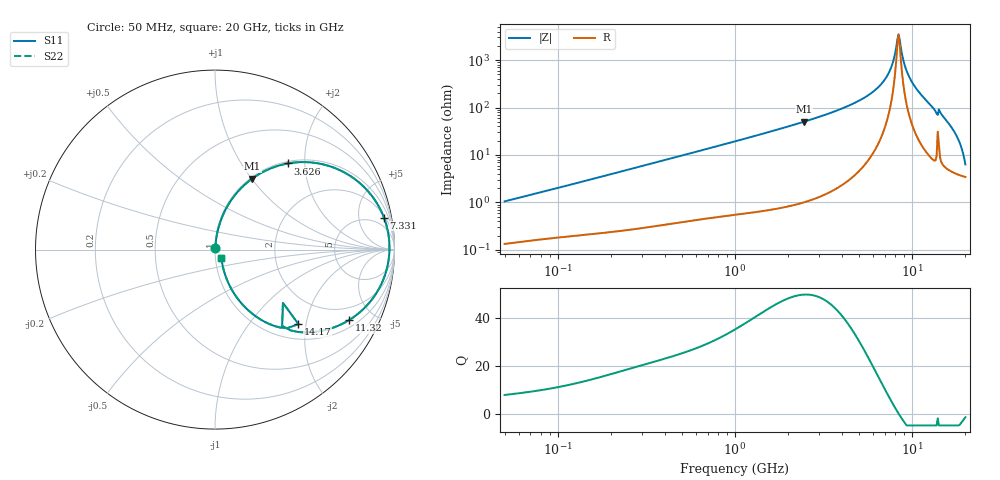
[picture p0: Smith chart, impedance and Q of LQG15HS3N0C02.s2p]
!Murata Part Number: LQG15HS3N0C02
!These Parameters are Measured in Series Mode Connection
!  o--[Z]--o
!Port1  Port2
!  o-------o
!Freq. Start=50[MHz] Stop=20[GHz], 401[Steps]
# Hz S RI R 50
!Freq.(Hz) S11(Real) S11(Imag) S21(Real) S21(Imag) S12(Real) S12(Imag) S22(Real) S22(Imag)
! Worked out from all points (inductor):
!   401 points, 50 MHz to 20 GHz, reference 50 ohm
!   read as one part in series: L = 3.28 nH near 51.52 MHz
!   highest Q = 50 at 2.456 GHz (marker M1), where L = 3.26 nH
!   self-resonance near 8.389 GHz
!   S11 on the Smith chart (normalised r, x): 50 MHz: 1.00, +0.02; 3.626 GHz: 1.04, +1.64; 7.331 GHz: 2, +10; 11.32 GHz: 1.32, -3.61; 14.17 GHz: 1.33, -1.81; 20 GHz: 1.07, -0.11
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5e7  0.00144 0.0104  0.9986 -0.0104  0.9986 -0.0104  0.00144 0.0104
1.364002e8  0.00278 0.0271  0.9972 -0.0271  0.9972 -0.0271  0.00278 0.0271
3.721004e8  0.00844 0.0718  0.9916 -0.0718  0.9916 -0.0718  0.00844 0.0718
1e9  0.0411 0.1848  0.9589 -0.1848  0.9589 -0.1848  0.0411 0.1848
2.456456e9  0.2071 0.3953  0.7929 -0.3953  0.7929 -0.3953  0.2071 0.3953
2.728004e9  0.2494 0.4228  0.7506 -0.4228  0.7506 -0.4228  0.2494 0.4228
3.626126e9  0.4047 0.4798  0.5953 -0.4798  0.5953 -0.4798  0.4047 0.4798
5.683258e9  0.7628 0.4044  0.2372 -0.4044  0.2372 -0.4044  0.7628 0.4044
6.601595e9  0.8802 0.2909  0.1198 -0.2909  0.1198 -0.2909  0.8802 0.2909
7.331367e9  0.9412 0.1784  0.0588 -0.1784  0.0588 -0.1784  0.9412 0.1784
7.442007e9  0.9477 0.1603  0.0523 -0.1603  0.0523 -0.1603  0.9477 0.1603
7.784049e9  0.9629 0.103  0.0371 -0.103  0.0371 -0.103  0.9629 0.103
8.264682e9  0.9719 0.0212  0.0281 -0.0212  0.0281 -0.0212  0.9719 0.0212
8.389408e9  0.972 2.59e-05  0.028 -2.59e-05  0.028 -2.59e-05  0.972 2.59e-05
9.457416e9  0.9353 -0.1731  0.0647 0.1731  0.0647 0.1731  0.9353 -0.1731
1.131968e10  0.7481 -0.3921  0.2519 0.3921  0.2519 0.3921  0.7481 -0.3921
1.295331e10  0.5202 -0.4612  0.4798 0.4612  0.4798 0.4612  0.5202 -0.4612
1.417136e10  0.4647 -0.4148  0.5353 0.4148  0.5353 0.4148  0.4647 -0.4148
1.504638e10  0.3034 -0.415  0.6966 0.415  0.6966 0.415  0.3034 -0.415
1.747767e10  0.1078 -0.2471  0.8922 0.2471  0.8922 0.2471  0.1078 -0.2471
1.855685e10  0.0639 -0.1612  0.9361 0.1612  0.9361 0.1612  0.0639 -0.1612
2e10  0.0359 -0.0494  0.9641 0.0494  0.9641 0.0494  0.0359 -0.0494
